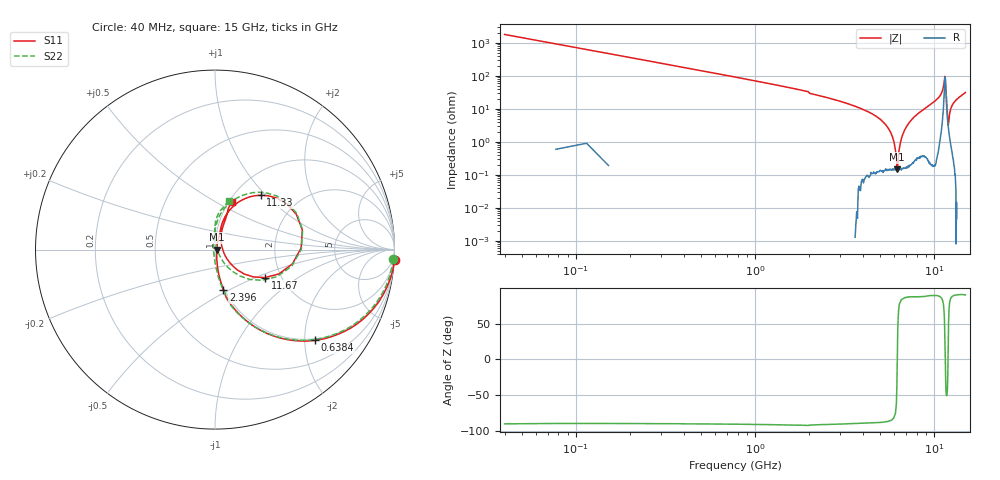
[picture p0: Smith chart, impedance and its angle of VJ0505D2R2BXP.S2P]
! VJ0505D2R2BXP
! MLCC placed on 25 mil thick microstrip substrate in series configuraton.
! DATE 06/29/2018  07:35
! CORRECTED  DATA
# GHz  S  MA  R  50.00
!  FREQ  S11M  S11A  S21M  S21A  S12M  S12A  S22M  S22A
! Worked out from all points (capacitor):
!   401 points, 40 MHz to 15 GHz, reference 50 ohm
!   read as one part in series: C = 2.22 pF near 114.8 MHz
!   lowest |Z| = 145 mohm at 6.248 GHz (marker M1)
!   series resonance near 6.244 GHz, so ESL is about 290 pH
!   S11 on the Smith chart (normalised r, x): 40 MHz: -1, -35; 638.4 MHz: 0.96, -2.23; 2.396 GHz: 0.99, -0.47; 11.33 GHz: 1.30, +0.94; 11.67 GHz: 1.65, -0.57; 15 GHz: 1.04, +0.60
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0.04  1.002 -3.3  0.05607 87.3  0.05625 87.3  0.9944 -3.2
0.2644  0.9425 -20.4  0.3471 69.8  0.3475 69.8  0.9348 -20.3
0.6384  0.7512 -42.3  0.6732 48.5  0.6732 48.5  0.7457 -42.2
1.3116  0.4715 -63.6  0.8964 28.1  0.897 28.1  0.4704 -63.7
2.3962  0.2288 -78.3  0.9788 13.3  0.9796 13.3  0.2294 -78.5
2.5458  0.2102 -78.9  0.9818 12.2  0.9823 12.2  0.2114 -79.5
5.0516  0.04693 -78.1  0.9969 2.6  0.9975 2.7  0.0467 -94.3
6.2484  0.009938 1.5  0.9977 -0.0  0.9983 0.0  0.008032 179.7
6.9216  0.02604 63.4  0.9975 -1.5  0.9978 -1.4  0.02464 109.7
7.52  0.04684 71.7  0.996 -2.8  0.9966 -2.7  0.04622 98.9
10.0258  0.1542 74.9  0.9844 -9.4  0.9856 -9.4  0.158 85.4
10.9608  0.2542 67.9  0.9488 -15.5  0.9491 -15.5  0.261 73.8
11.3348  0.3958 49.9  0.8161 -23.5  0.8166 -23.5  0.403 52.5
11.5218  0.4989 12.8  0.5273 -13.7  0.5278 -13.7  0.5004 12.6
11.6714  0.3193 -29.2  0.7426 11.4  0.7429 11.4  0.3137 -33.1
11.8584  0.1081 -41.3  0.9333 3.5  0.9336 3.5  0.09285 -55.9
11.9706  0.05378 -21.4  0.9629 0.1  0.9637 0.1  0.02838 -46.0
12.0454  0.04173 9.0  0.9726 -1.5  0.9732 -1.5  0.01215 36.2
12.2698  0.06775 60.6  0.9843 -4.7  0.9848 -4.7  0.06425 90.4
12.5316  0.1024 69.1  0.9872 -6.9  0.9879 -6.9  0.1047 91.0
13.2796  0.1666 70.8  0.9836 -10.9  0.9841 -10.9  0.1719 87.7
15  0.2812 70.2  0.9571 -18.2  0.9573 -18.2  0.2834 74.1
